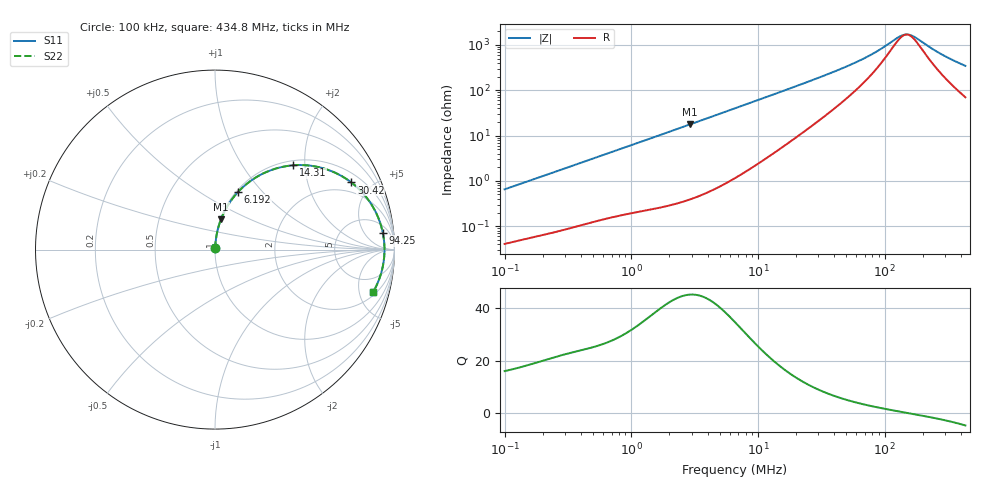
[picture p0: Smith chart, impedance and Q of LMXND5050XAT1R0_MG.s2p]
! LMXND5050XAT1R0_MG  S-PARAMETER MODEL  ( General Type )
! Model Generated by TAIYO YUDEN Corporation (http://www.ty-top.com)
! Version 1.0
! TAIYO YUDEN Control No. 191023NI43SB-FBB
! Copyright(c) 2019 TAIYO YUDEN CO.,LTD. All Rights Reserved.
! Product Description (link to TY-COMPAS)
! https://ds.yuden.co.jp/TYCOMPAS/or/detail?pn=LMXND5050XAT1R0NMG&u=M
! Products Name : Inductors
! Characteristics :
!  Inductance : 1.0 uH , SRF(min) : 110 MHz , DC Resistance(max) : 0.0195 Ohm
!  Rated Current : Saturation :6600 mA , Temp Rise : 4000 mA
!  Case Size : 4.9 x 4.9 / 0.193 x 0.193 [mm/inch] , Thickness : 3.1 / 0.122 [mm/inch]
!  (Conditions: Temperature = 25 degC , DC Bias Current/Voltage = 0A / 0V)
! External Node Assignments :
!  1  o---GGG---o  2
! GND o---------o GND
! Frequency Range : 0.1MHz  -  434.768421MHz  [ 402 STEP ]
# MHz S RI R 50
! Freq[MHz].  S11 Real  S11 Imag  S21 Real  S21 Imag  S12 Real  S12 Imag  S22 Real  S22 Imag
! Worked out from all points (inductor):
!   401 points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, 100 kHz to 434.8 MHz, reference 50 ohm
!   read as one part in series: L = 1.02 uH near 104.3 kHz
!   highest Q = 45.3 at 2.913 MHz (marker M1), where L = 962 nH
!   self-resonance near 149.5 MHz
!   S11 on the Smith chart (normalised r, x): 100 kHz: 1.00, +0.01; 6.192 MHz: 1.02, +0.75; 14.31 MHz: 1.09, +1.74; 30.42 MHz: 1.43, +3.78; 94.25 MHz: 9, +14; 434.8 MHz: 2.40, -6.75
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0.1  0.000447 0.00648  0.9996 -0.00648  0.9996 -0.00648  0.000447 0.00648
0.406826  0.0017 0.0253  0.9983 -0.0253  0.9983 -0.0253  0.0017 0.0253
1.65507  0.0124 0.0989  0.9876 -0.0989  0.9876 -0.0989  0.0124 0.0989
2.913391  0.0336 0.1695  0.9664 -0.1695  0.9664 -0.1695  0.0336 0.1695
4.429062  0.0719 0.2468  0.9281 -0.2468  0.9281 -0.2468  0.0719 0.2468
6.192158  0.1296 0.3223  0.8704 -0.3223  0.8704 -0.3223  0.1296 0.3223
6.733248  0.1493 0.3421  0.8507 -0.3421  0.8507 -0.3421  0.1493 0.3421
9.612815  0.261 0.4206  0.739 -0.4206  0.739 -0.4206  0.261 0.4206
14.31093  0.4345 0.4695  0.5655 -0.4695  0.5655 -0.4695  0.4345 0.4695
19.18699  0.5744 0.4602  0.4256 -0.4602  0.4256 -0.4602  0.5744 0.4602
26.82484  0.7158 0.4039  0.2842 -0.4039  0.2842 -0.4039  0.7158 0.4039
30.41663  0.7593 0.3743  0.2407 -0.3743  0.2407 -0.3743  0.7593 0.3743
40.78027  0.8384 0.2977  0.1616 -0.2977  0.1616 -0.2977  0.8384 0.2977
57.01386  0.895 0.2099  0.105 -0.2099  0.105 -0.2099  0.895 0.2099
94.24882  0.935 0.0936  0.065 -0.0936  0.065 -0.0936  0.935 0.0936
109.1303  0.9402 0.063  0.0598 -0.063  0.0598 -0.063  0.9402 0.063
137.4034  0.9441 0.0167  0.0559 -0.0167  0.0559 -0.0167  0.9441 0.0167
149.4101  0.9444 0.000131  0.0556 -0.000131  0.0556 -0.000131  0.9444 0.000131
159.0988  0.9443 -0.0123  0.0557 0.0123  0.0557 0.0123  0.9443 -0.0123
176.6629  0.9433 -0.0331  0.0567 0.0331  0.0567 0.0331  0.9433 -0.0331
280.0589  0.9262 -0.1299  0.0738 0.1299  0.0738 0.1299  0.9262 -0.1299
434.7684  0.881 -0.2365  0.119 0.2365  0.119 0.2365  0.881 -0.2365
